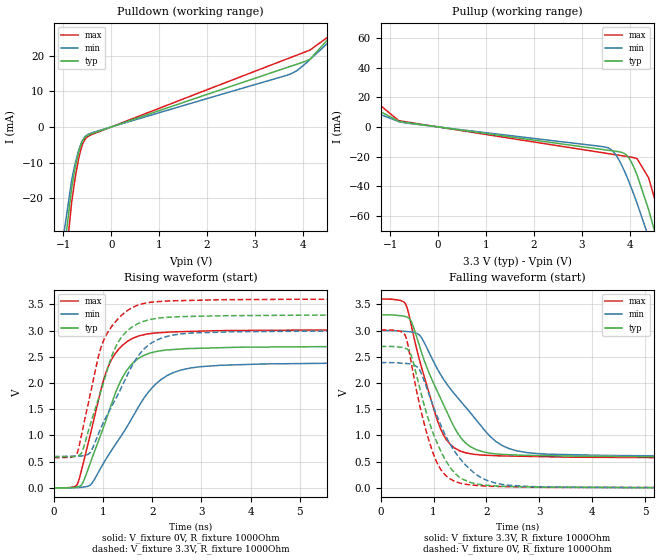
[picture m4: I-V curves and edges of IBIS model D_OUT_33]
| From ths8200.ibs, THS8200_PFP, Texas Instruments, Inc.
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[Model]   D_OUT_33
Model_type   Output
Polarity   Non-Inverting
Vmeas = 1.65
Vref = 1.65
Cref = 15pF
Rref = 1000
|   typ   min   max
C_comp   1.273p   1.273p   1.273p
[Voltage Range]   3.3   3   3.6
[Temperature Range]   27   85   0
[Pullup Reference]   3.3   3   3.6
[Pulldown Reference]   -0   -0   -0
[Power Clamp Reference]   3.3   3   3.6
[GND Clamp Reference]   -0   -0   -0
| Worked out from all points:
|   slope of the pulldown table from 0 to 0.495 V, typ, clamps not added: 218 ohm
|   slope of the pullup table from 0 to 0.495 V, typ, clamps not added: 224 ohm
|   falling waveform, V_fixture 3.3V, R_fixture 1000Ohm: 20-80 % time 687ps typ, 1.04ns min, 510ps max; typ from 3.3 V to 0.589 V
|   rising waveform, V_fixture 0V, R_fixture 1000Ohm: 20-80 % time 662ps typ, 985ps min, 521ps max; typ from 0 V to 2.7 V
|   rising waveform, V_fixture 3.3V, R_fixture 1000Ohm: 20-80 % time 579ps typ, 790ps min, 516ps max; typ from 0.589 V to 3.3 V
|   falling waveform, V_fixture 0V, R_fixture 1000Ohm: 20-80 % time 544ps typ, 700ps min, 438ps max; typ from 2.7 V to 0 V
[Pulldown]
|   Voltage   I(typ)   I(min)   I(max)
-3.3V     -1.546A    -1.457A    -1.589A
-1.657V   -110.7mA   -91.37mA   -128.9mA
-825mV    -16.91mA   -14.72mA   -20.87mA
-726mV    -9.68mA    -8.74mA    -12.12mA
-636.9mV  -5.155mA   -4.862mA   -6.413mA
-557.7mV  -3.088mA   -2.913mA   -3.669mA
-458.7mV  -2.149mA   -1.925mA   -2.462mA
3.749V    17.04mA    14.9mA     19.5mA
3.887V    17.66mA    15.94mA    20.22mA
4.145V    18.96mA    18.86mA    21.54mA
4.66V     26.63mA    25.32mA    26.59mA
6.59V     60.68mA    50.09mA    80.13mA
[Pullup]
|   Voltage   I(typ)   I(min)   I(max)
-3.3V     46.15mA    35mA       70.57mA
-825mV    3.825mA    3.575mA    4.269mA
3.531V    -15.65mA   -13.94mA   -17.89mA
3.61V     -16mA      -15.26mA   -18.28mA
3.719V    -16.49mA   -19.3mA    -18.83mA
3.887V    -17.95mA   -29.74mA   -19.68mA
3.986V    -21.23mA   -37.33mA   -20.18mA
4.075V    -26.57mA   -44.78mA   -20.68mA
4.155V    -32.7mA    -51.79mA   -21.48mA
4.392V    -55.72mA   -74.38mA   -34.29mA
4.749V    -96.97mA   -112.5mA   -74.17mA
6.59V     -1.537A    -1.741A    -1.285A
[Ramp]
R_load = 1000
|   typ   min   max
dV/dt_r   1.61874/6.62249e-10   1.43327/9.85946e-10   1.80679/5.20601e-10
dV/dt_f   1.62657/6.8717e-10   1.44085/1.03644e-09   1.8151/5.09842e-10
[Falling Waveform]
V_fixture = 3.3V
V_fixture_min = 3V
V_fixture_max = 3.6V
R_fixture = 1000Ohm
C_fixture = 0F
|   Time   V(typ)   V(min)   V(max)
0s        3.3V       3V         3.6V
473ps     3.266V     2.983V     3.501V
579.9ps   3.17V      2.974V     3.095V
745.3ps   2.669V     2.899V     2.395V
1.138ns   1.695V     2.153V     1.112V
1.308ns   1.327V     1.903V     836.7mV
1.608ns   856.1mV    1.537V     667.5mV
2.179ns   648.3mV    884.5mV    613.1mV
2.775ns   620.4mV    671.6mV    600.6mV
10ns      589.1mV    598.6mV    574.8mV
[Rising Waveform]
V_fixture = 0V
V_fixture_min = 0V
V_fixture_max = 0V
R_fixture = 1000Ohm
C_fixture = 0F
|   Time   V(typ)   V(min)   V(max)
0s        1.51nV     5.749nV    1.328nV
453.2ps   14.28mV    4.319mV    39.2mV
567.4ps   60.96mV    10.8mV     354.1mV
761ps     526mV      71.39mV    1.093V
1.138ns   1.503V     664.3mV    2.381V
1.411ns   2.131V     1.051V     2.731V
1.738ns   2.478V     1.573V     2.902V
2.304ns   2.631V     2.143V     2.969V
2.969ns   2.663V     2.31V      2.989V
10ns      2.698V     2.389V     3.011V
[Rising Waveform]
V_fixture = 3.3V
V_fixture_min = 3V
V_fixture_max = 3.6V
R_fixture = 1000Ohm
C_fixture = 0F
|   Time   V(typ)   V(min)   V(max)
0s        589mV      597.8mV    574.8mV
463.1ps   607.4mV    605.5mV    637.8mV
567.4ps   674.4mV    608.7mV    1.029V
729.5ps   1.171V     663.2mV    1.738V
909.4ps   1.706V     1.035V     2.514V
1.054ns   2.147V     1.339V     2.895V
1.313ns   2.788V     1.799V     3.233V
1.738ns   3.145V     2.545V     3.497V
2.775ns   3.27V      2.953V     3.575V
10ns      3.3V       2.999V     3.6V
[Falling Waveform]
|Gnd
V_fixture = 0V
V_fixture_min = 0V
V_fixture_max = 0V
R_fixture = 1000Ohm
C_fixture = 0F
|   Time   V(typ)   V(min)   V(max)
0s        2.698V     2.39V      3.011V
422ps     2.677V     2.377V     2.962V
542.4ps   2.602V     2.367V     2.583V
745.3ps   1.874V     2.229V     1.539V
1.017ns   975.3mV    1.493V     589.8mV
1.239ns   505.7mV    972.7mV    227.1mV
1.501ns   196.9mV    557mV      89.78mV
1.916ns   58.45mV    185.5mV    39.53mV
2.429ns   25.94mV    48.91mV    22.8mV
10ns      30.33uV    221.8uV    2.983uV
